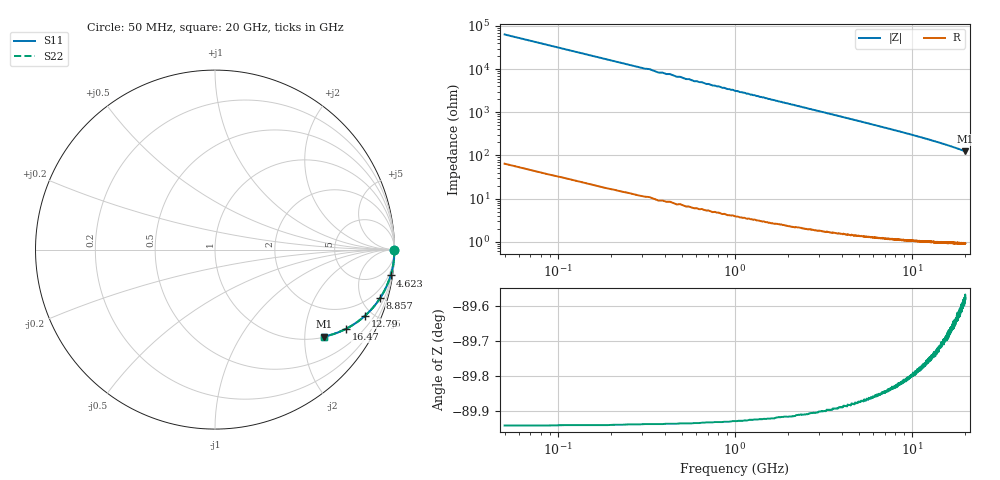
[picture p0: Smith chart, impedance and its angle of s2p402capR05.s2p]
! AVX Thin Film Operation		Date: September 2011
! Description: Accu-P® Series, Thin Film, SMD, RF Capacitor
! Part Number: 04021JR05ZBW/STR
! 50 MHz  -  20 GHz
! Serial Measurements
# MHZ S MA R 50
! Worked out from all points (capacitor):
!   1000 points, 50 MHz to 20 GHz, reference 50 ohm
!   read as one part in series: C = 50 fF near 149.8 MHz
!   lowest |Z| = 124 ohm at 20 GHz (marker M1)
!   S11 on the Smith chart (normalised r, x): 50 MHz: open; 4.623 GHz: 1, -14; 8.857 GHz: 1.03, -6.88; 12.79 GHz: 1.02, -4.53; 16.47 GHz: 1.02, -3.29; 20 GHz: 1.02, -2.48
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50  1 -0.1  0.001571 89.9  0.001571 89.9  1 -0.1
89.94  1 -0.2  0.002826 89.8  0.002826 89.8  1 -0.2
169.82  1 -0.3  0.005335 89.6  0.005335 89.6  1 -0.3
209.76  1 -0.4  0.00659 89.6  0.00659 89.6  1 -0.4
309.61  1 -0.6  0.009727 89.4  0.009727 89.4  1 -0.6
429.429  1 -0.8  0.013 89.2  0.013 89.2  1 -0.8
549.249  1 -1.0  0.017 88.9  0.017 88.9  1 -1.0
689.039  1 -1.2  0.022 88.7  0.022 88.7  1 -1.2
848.799  1 -1.5  0.027 88.4  0.027 88.4  1 -1.5
1308.108  0.999 -2.4  0.041 87.6  0.041 87.6  0.999 -2.4
1847.297  0.998 -3.3  0.058 86.6  0.058 86.6  0.998 -3.3
2586.186  0.997 -4.7  0.081 85.2  0.081 85.2  0.997 -4.7
3384.985  0.994 -6.1  0.106 83.8  0.106 83.8  0.994 -6.1
4623.123  0.989 -8.4  0.145 81.5  0.145 81.5  0.989 -8.4
6700  0.977 -12.2  0.211 77.7  0.211 77.7  0.977 -12.2
8856.757  0.959 -16.2  0.279 73.6  0.279 73.6  0.959 -16.2
10034.99  0.948 -18.4  0.316 71.4  0.316 71.4  0.948 -18.4
12790.84  0.913 -23.8  0.403 66.0  0.403 66.0  0.913 -23.8
13350  0.905 -24.9  0.421 64.8  0.421 64.8  0.905 -24.9
16465.31  0.852 -31.2  0.518 58.5  0.518 58.5  0.852 -31.2
16684.99  0.848 -31.7  0.525 58.0  0.525 58.0  0.848 -31.7
20000  0.776 -38.7  0.625 50.9  0.625 50.9  0.776 -38.7
